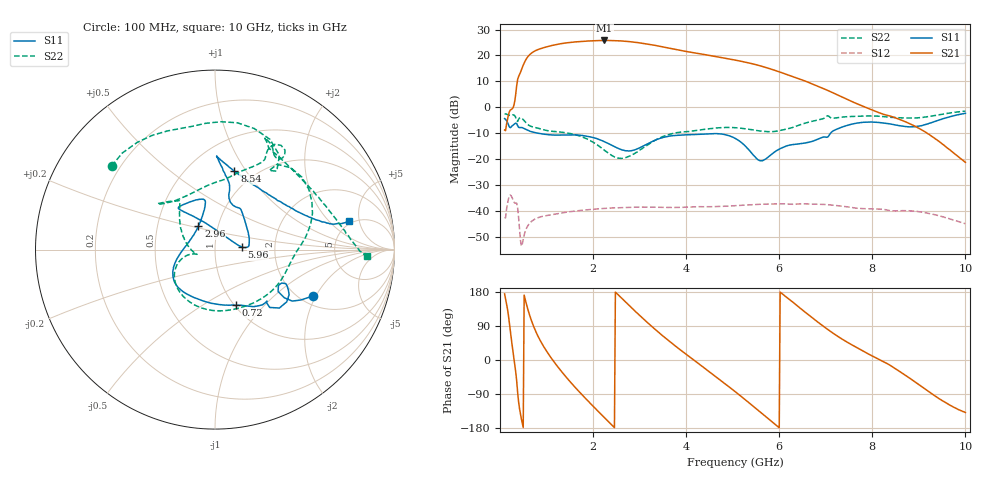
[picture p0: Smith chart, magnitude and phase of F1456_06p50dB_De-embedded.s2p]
! Integrated Device Technology
! Corporate Headquarters
! 6024 Silver Creek Valley Road
! San Jose, CA 95138  USA
! Phone:  1-408-284-8200
! Toll Free:  1-800-223-1366
! Webpage:  http://www.idt.com/
! Timing and RF Division
! 515 Groton Road, Suite 102
! Westford, MA 01886-6024
! Device:  F1456
! Description: 6-bit 0.5 dB Transmit Variable Gain Amplifier
! Frequency:  2100.0 -  2950.00 MHz
! Package:  6x6 mm Thin QFN Plastic Package: 28 pin
! State:  13
! Atten State:  6.5 dB
! Voltage:  +5.00 Volts
! Current:  217.046 mA
! Data:  The device was measured on a the F1455 evaluation board which has
!  individual transmission lines to the RF pins.  Data was collected
!  using a calibrated network analyzer.  The evaluation board was
!  de-embedded using a TRL calibration technique.
!  The reference plane is the edge of the package pin.
!  Pin  1 = CSb
!  Pin  2 = DATA
!  Pin  3 = CLK
!  Pin  4 = RSET
!  Pin  5 = GND
!  Pin  6 = RFIN  = Port 1
!  Pin  7 = GND
!  Pin  8 = NC
!  Pin  9 = NC
!  Pin 10 = NC
!  Pin 11 = NC
!  Pin 12 = NC
!  Pin 13 = NC
!  Pin 14 = /STBY
!  Pin 15 = GND
!  Pin 16 = RFOUT  = Port 2
!  Pin 17 = GND
!  Pin 18 = NC
!  Pin 19 = NC
!  Pin 20 = NC
!  Pin 21 = GND
!  Pin 22 = NC
!  Pin 23 = GND
!  Pin 24 = NC
!  Pin 25 = NC
!  Pin 26 = NC
!  Pin 27 = GND
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# GHz S dB R 50
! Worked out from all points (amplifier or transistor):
!   496 points, 100 MHz to 10 GHz, reference 50 ohm
!   highest |S21| = 25.8 dB at 2.24 GHz (marker M1)
!   |S21| within 3 dB of that: 900.2 MHz to 3.645 GHz (2.745 GHz wide, 121 % of centre)
!   unconditionally stable (mu >= 1): start of sweep to end of sweep
!   at 1.74 GHz: K = 2.37, MAG = 26.0 dB, |S12| = -39.8 dB
!   at 5.06 GHz: K = 3.93, MAG = 19.2 dB, |S12| = -37.9 dB
!   at 10 GHz: K = 119.90, MAG = -12.0 dB, |S12| = -44.9 dB
!   S11 on the Smith chart (normalised r, x): 100 MHz: 2.35, -1.90; 720 MHz: 1.01, -0.71; 2.96 GHz: 0.80, +0.21; 5.96 GHz: 1.35, +0.04; 8.54 GHz: 0.81, +0.89; 10 GHz: 4.66, +3.61
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0.1  -4.36 -25.1  -8.76 174.4  -42.50 44.4  -2.61 141.1
0.34  -6.12 -36.1  5.22 -32.6  -36.93 -145.9  -3.93 55.6
0.42  -7.80 -44.7  12.61 -128.2  -46.84 137.7  -4.13 47.2
0.56  -8.52 -57.6  18.47 151.4  -47.06 -174.1  -5.95 6.9
0.72  -9.59 -69.5  21.43 89.8  -43.45 140.7  -7.64 -16.2
0.96  -10.40 -90.5  23.10 31.4  -41.88 93.2  -8.76 -55.5
1.18  -10.72 -108.8  24.10 -7.9  -41.21 66.8  -9.33 -87.2
1.5  -10.63 -129.3  25.01 -56.3  -40.26 38.7  -10.07 -125.2
1.76  -10.83 -142.5  25.43 -91.3  -39.71 20.2  -11.36 -146.9
2.24  -13.20 -166.3  25.79 -151.5  -38.99 -9.1  -16.47 -168.8
2.58  -16.11 167.4  25.63 167.1  -38.68 -28.1  -19.68 -165.3
2.96  -15.96 125.6  24.97 122.4  -38.51 -48.2  -17.01 177.0
3.4  -12.25 103.3  23.66 73.9  -38.53 -70.0  -12.11 141.8
3.74  -10.89 102.5  22.45 39.6  -38.63 -84.6  -9.98 128.1
4.1  -10.55 113.0  21.23 6.0  -38.46 -99.3  -9.22 128.4
4.6  -10.12 130.1  19.69 -40.6  -38.31 -120.7  -8.05 138.7
5.06  -12.03 127.0  18.19 -84.1  -37.94 -140.0  -7.87 141.2
5.96  -16.53 5.7  13.94 -174.7  -37.21 172.5  -9.14 102.7
6.7  -13.18 37.5  9.12 112.3  -37.26 128.4  -5.43 63.1
8.36  -6.34 83.2  -3.27 -12.2  -39.79 52.2  -3.82 62.4
8.54  -6.92 76.1  -4.33 -26.5  -39.89 47.7  -3.99 58.0
10  -2.32 12.1  -21.21 -138.5  -44.90 -31.4  -1.46 -2.5
